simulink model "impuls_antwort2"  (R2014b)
settings: Solver=ode5  StartTime=0.0  StopTime=20.0  MaxStep=0.001  RelTol=1e-3
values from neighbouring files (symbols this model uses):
  C = [0 1 0 0;0 0 0 1]    [impuls_antw_zustand_1.m]    (also in impuls_antwort_1.m = 1e-07; impuls_antwort_2.m = 1e-07; impuls_antwort_3.m = 1e-07; impuls_antwort_4.m = 1e-07)
  L = 0.01    [impuls_antwort_1.m]    (also in impuls_antwort_2.m; impuls_antwort_3.m; impuls_antwort_4.m; RLC_reihen_1.m)
  R = 50    [impuls_antwort_1.m]    (also in impuls_antwort_2.m; impuls_antwort_3.m; impuls_antwort_4.m; RLC_reihen_1.m)

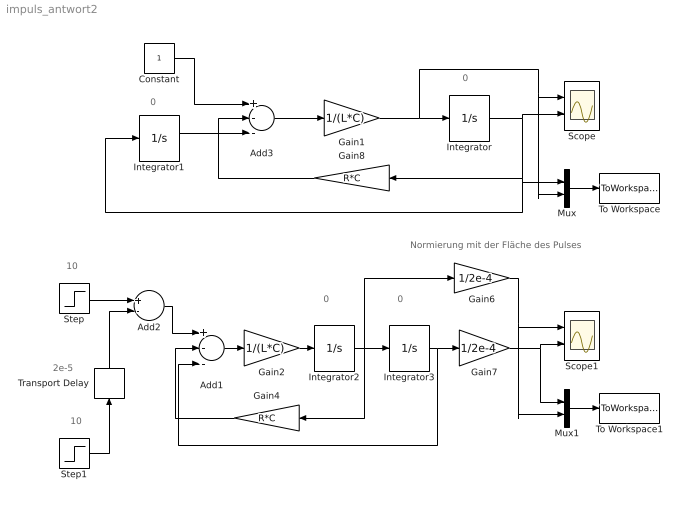
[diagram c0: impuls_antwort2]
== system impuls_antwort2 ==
  note: Normierung mit der Fläche des Pulses
  note: 2e-5
  note: 0
  note: 0
  note: 10
  note: 10
  note: 0
  note: 0
  Add1 : Sum  Inputs=+--
  Add2 : Sum  Inputs=+-
  Add3 : Sum  Inputs=+--
  Constant : Constant
  Gain1 : Gain  Gain=1/(L*C)
  Gain2 : Gain  Gain=1/(L*C)
  Gain4 : Gain  Gain=R*C
  Gain6 : Gain  Gain=1/2e-4
  Gain7 : Gain  Gain=1/2e-4
  Gain8 : Gain  Gain=R*C
  Integrator{,1..3} (4 alike) : Integrator
  Mux : Mux  Inputs=2
  Mux1 : Mux  Inputs=2
  Scope : Scope  NumInputPorts=2
  Scope1 : Scope  NumInputPorts=2
  Step : Step  Time=0  After=10  SampleTime=0
  Step1 : Step  Time=0  After=10  SampleTime=0
  To Workspace : ToWorkspace  VariableName=simout  SaveFormat=Timeseries  SampleTime=-1
  To Workspace1 : ToWorkspace  VariableName=simout1  SaveFormat=Timeseries  SampleTime=-1
  Transport Delay : TransportDelay  DelayTime=2e-5
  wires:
  Gain2/1 -> Integrator2/1
  Integrator2/1 -> Gain4/1, Integrator3/1, Gain6/1
  Integrator3/1 -> Add1/3, Gain7/1
  Gain4/1 -> Add1/2
  Step/1 -> Add2/1
  Step1/1 -> Transport Delay/1
  Add2/1 -> Add1/1
  Transport Delay/1 -> Add2/2
  Gain6/1 -> Mux1/2, Scope1/1
  Gain7/1 -> Mux1/1, Scope1/2
  Add3/1 -> Gain1/1
  Gain1/1 -> Mux/2, Scope/1, Integrator/1
  Integrator/1 -> Scope/2, Mux/1, Integrator1/1, Gain8/1
  Constant/1 -> Add3/1
  Add1/1 -> Gain2/1
  Gain8/1 -> Add3/2
  Integrator1/1 -> Add3/3
  Mux/1 -> To Workspace/1
  Mux1/1 -> To Workspace1/1
